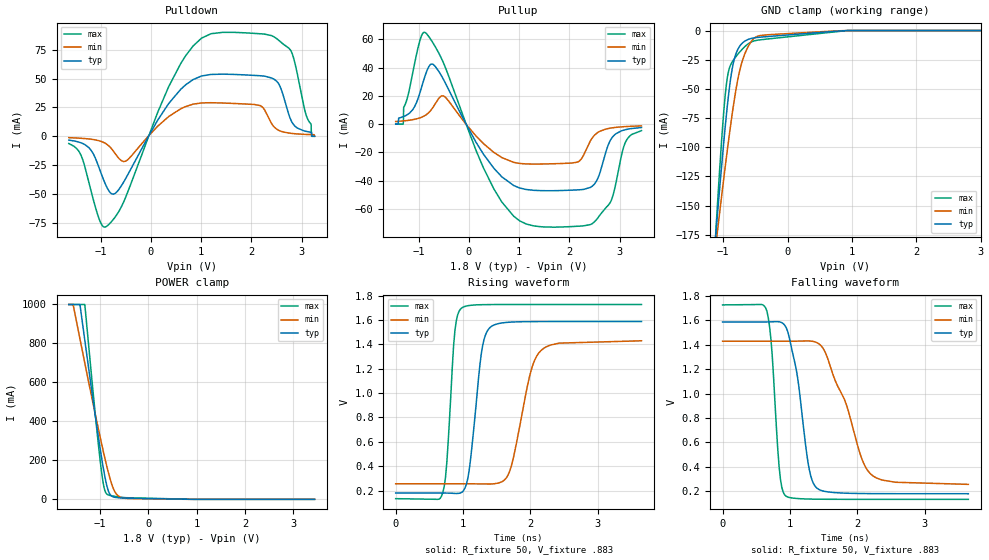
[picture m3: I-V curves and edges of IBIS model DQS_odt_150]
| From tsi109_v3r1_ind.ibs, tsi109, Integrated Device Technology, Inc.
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|   MODEL DQS_odt_150
[Model]   DQS_odt_150
Model_type  I/O
Polarity   Non-Inverting
Enable   Active-Low
|   typ   min   max
|C_comp_off 3.705p 3.718p 3.636p
|C_comp_on 3.3p 3.146p 3.514p
C_comp 3.503p 3.432p 3.575p
Cref  =   20pF
Vmeas =   0.9v
Vinl  =   0.650v
Vinh  =   1.150v
[Model Spec]
[Temperature Range]   25   125   -40
[Voltage Range] 1.8 1.71 1.89
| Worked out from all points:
|   slope of the pulldown table from 0 to 0.27 V, typ, clamps not added: 14.1 ohm
|   slope of the pullup table from 0 to 0.27 V, typ, clamps not added: 16.4 ohm
|   rising waveform, R_fixture 50, V_fixture .883: 20-80 % time 155ps typ, 260ps min, 101ps max; typ from 0.179 V to 1.59 V
|   falling waveform, R_fixture 50, V_fixture .883: 20-80 % time 210ps typ, 436ps min, 109ps max; typ from 1.59 V to 0.179 V
[Pulldown]
-1.636V   -3.323mA   -1.212mA   -6.261mA
-1.394V   -5.682mA   -1.723mA   -16.41mA
-1.201V   -11.61mA   -2.501mA   -46.1mA
-1.012V   -29.76mA   -4.157mA   -73.79mA
-864mV    -45.35mA   -7.415mA   -77.34mA
-502.6mV  -36.5mA    -21.48mA   -52.62mA
591.4mV   40.58mA    23.75mA    62.85mA
1.433V    53.78mA    28.8mA     89.99mA
2.176V    52.4mA     26.59mA    88.74mA
2.463V    49.07mA    7.654mA    85.76mA
2.755V    17.73mA    2.744mA    75.92mA
3.26V     0A         0A         0A
[Pullup]
-1.46V    0A         1.84mA     0A
-1.311V   5.209mA    2.254mA    0A
-1.301V   5.351mA    2.288mA    11.66mA
-875.5mV  33.99mA    6.09mA     64.83mA
-504.2mV  31.36mA    19.84mA    42.99mA
495.7mV   -31.23mA   -20.01mA   -45.83mA
1.456V    -47.09mA   -28.22mA   -72.68mA
2.164V    -46.52mA   -26.87mA   -72.25mA
2.496V    -42.58mA   -8.056mA   -69.28mA
2.862V    -9.049mA   -2.593mA   -51.25mA
3.119V    -3.923mA   -1.743mA   -12.68mA
3.436V    -2.406mA   -1.258mA   -4.612mA
[GND Clamp]
-1.636V   -544mA     -441.4mA   -698.5mA
-1.119V   -177.5mA   -186.1mA   -176.7mA
-1.104V   -167.6mA   -179.1mA   -162.9mA
-1.079V   -151.2mA   -167.4mA   -140.4mA
-1.004V   -103.8mA   -133mA     -79.08mA
-934.4mV  -64.27mA   -102.2mA   -40.21mA
-824.9mV  -24.2mA    -58.74mA   -24.08mA
-745.3mV  -13.62mA   -34.97mA   -18.58mA
-660.7mV  -9.028mA   -19.65mA   -13.68mA
-521.3mV  -6.307mA   -6.754mA   -8.964mA
-307.3mV  -5.162mA   -3.62mA    -7.232mA
3.26V     0A         0A         0A
[Power Clamp]
-1.636V   1A         1A         1A
-1.546V   1A         997.3mA    1A
-1.407V   998.2mA    823.6mA    1A
-1.307V   817.6mA    699.9mA    1A
-1.093V   433.9mA    439.6mA    442.1mA
-982.8mV  250.1mA    311.6mA    185.5mA
-913mV    144.8mA    233.7mA    66.23mA
-848.2mV  66.74mA    165.6mA    26.32mA
-783.3mV  24.69mA    104.6mA    19.92mA
-688.6mV  10.68mA    40.26mA    15.37mA
-494mV    6.246mA    5.746mA    9.037mA
3.436V    0A         0A         0A
[Ramp]
dV/dt_r .845/154.678p .705/260.261p .956/101.167p
dV/dt_f .845/210.589p .705/436.081p .956/108.694p
[Rising Waveform]
R_fixture = 50
V_fixture = .883
V_fixture_min = .842
V_fixture_max = .93
0s        179.2mV    255.2mV    133.3mV
690ps     179.3mV    255.2mV    168.3mV
760ps     179mV      255.2mV    435.5mV
880ps     176.2mV    255.2mV    1.514V
980ps     185.4mV    255.3mV    1.698V
1.29ns    1.386V     254.4mV    1.726V
1.41ns    1.542V     253.8mV    1.727V
1.69ns    1.582V     354.6mV    1.727V
2.15ns    1.587V     1.345V     1.727V
3.65ns    1.588V     1.429V     1.727V
[Falling Waveform]
R_fixture = 50
V_fixture = .883
V_fixture_min = .842
V_fixture_max = .93
0s        1.588V     1.429V     1.727V
660ps     1.588V     1.429V     1.674V
720ps     1.588V     1.429V     1.437V
840ps     1.589V     1.429V     399.9mV
940ps     1.545V     1.429V     160.3mV
1.11ns    1.147V     1.43V      140mV
1.29ns    371.6mV    1.431V     135.5mV
1.39ns    231.1mV    1.42V      134.5mV
2.21ns    180.2mV    336.1mV    133.3mV
3.65ns    179.2mV    256.1mV    133.3mV
